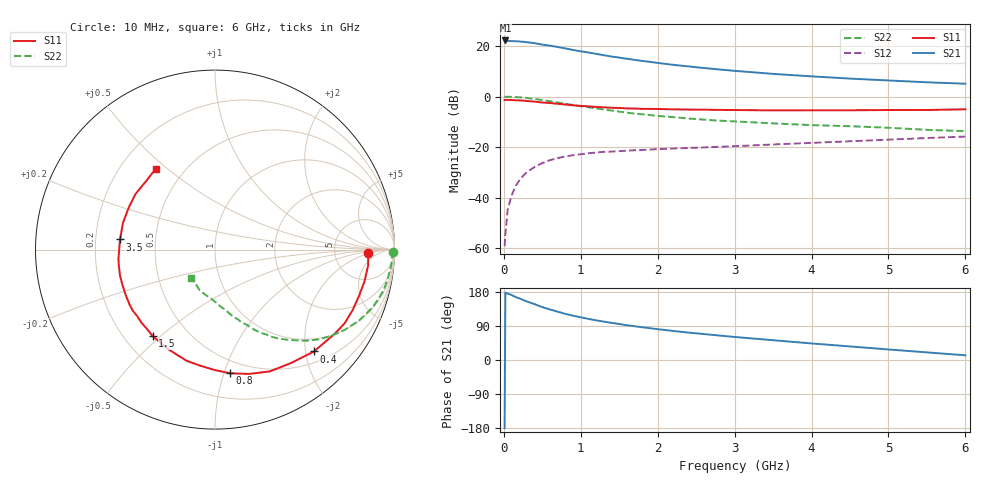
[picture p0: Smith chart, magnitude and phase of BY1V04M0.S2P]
! SIEMENS Small Signal Semiconductors
! BFY420
! Si NPN RF SIEGET Grounded Emitter Transistor in MICRO-X
! VCE = 1 V  IC = 4 mA
! Common Emitter S-Parameters:  October  1996
# GHz  S  MA  R  50
!  f  S11  S21  S12  S22
! GHz  MAG  ANG  MAG  ANG  MAG  ANG  MAG  ANG
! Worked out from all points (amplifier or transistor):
!   36 points, 10 MHz to 6 GHz, reference 50 ohm
!   highest |S21| = 22.2 dB at 20 MHz (marker M1)
!   |S21| within 3 dB of that: start of sweep to 772 MHz
!   unconditionally stable (mu >= 1): 3.283 GHz to end of sweep
!   at 250 MHz: K = 0.10, MSG = 26.5 dB, |S12| = -31.4 dB
!   at 1.4 GHz: K = 0.48, MSG = 18.8 dB, |S12| = -21.8 dB
!   at 6 GHz: K = 1.18, MAG = 7.8 dB, |S12| = -15.8 dB
!   S11 on the Smith chart (normalised r, x): 10 MHz: 13, -2; 400 MHz: 0.71, -2.17; 800 MHz: 0.39, -1.05; 1.5 GHz: 0.32, -0.47; 3.5 GHz: 0.31, +0.05; 6 GHz: 0.35, +0.46
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0.01  0.8552 -1.4  12.75 -179.9  0.0011 93.4  0.9909 -0.7
0.02  0.8541 -2.6  12.83 177.8  0.0019 95.1  0.9861 -1.3
0.05  0.8577 -5.9  12.53 175.1  0.0058 87.6  0.9886 -3.4
0.1  0.8516 -12.1  12.47 171.7  0.0109 84.4  0.9814 -7.0
0.15  0.8428 -17.8  12.38 166.3  0.0168 79.4  0.9741 -10.4
0.25  0.831 -29.6  12.07 158.4  0.027 73.3  0.9496 -17.0
0.3  0.8158 -35.0  11.85 154.3  0.0321 71.5  0.9351 -20.2
0.4  0.7914 -45.8  11.32 147.4  0.0404 65.2  0.8948 -26.2
0.5  0.761 -56.2  10.63 139.5  0.0484 60.6  0.8519 -31.5
0.6  0.7439 -65.9  10.12 133.4  0.0552 55.8  0.8077 -36.5
0.8  0.6945 -83.0  8.91 121.8  0.0655 48.3  0.7191 -44.9
0.9  0.6707 -90.2  8.316 116.9  0.0691 45.4  0.6795 -48.1
1.1  0.6395 -104.2  7.414 108.5  0.0756 40.5  0.6109 -54.3
1.3  0.6119 -115.7  6.555 101.3  0.0805 36.9  0.5522 -58.9
1.5  0.5936 -125.8  5.886 95.0  0.0831 34.2  0.5023 -63.4
1.8  0.5703 -139.4  5.044 86.4  0.0877 31.3  0.445 -68.2
2.2  0.5578 -153.4  4.234 76.7  0.0935 28.7  0.3913 -74.3
2.8  0.5438 -169.9  3.427 64.6  0.1015 26.7  0.3327 -81.6
3.5  0.5323 173.9  2.799 52.2  0.1126 24.8  0.2941 -89.2
4.5  0.5346 154.1  2.261 35.8  0.1304 20.9  0.2588 -101.4
5.5  0.5414 135.0  1.911 20.1  0.1511 16.0  0.2194 -119.5
6  0.5581 126.4  1.789 12.4  0.1615 12.9  0.2068 -130.6
